DATA_BLOCK DB 1
TITLE =
VERSION : 0.1


  STRUCT
   DB_VAR : BOOL ;	//vorläufige Platzhaltervariable
  END_STRUCT ;
BEGIN
   DB_VAR := FALSE;
END_DATA_BLOCK

DATA_BLOCK "Globaler DB10"
TITLE =
AUTHOR : 'Kleißler'
VERSION : 0.1


  STRUCT
   DB_VAR : INT ;	//vorläufige Platzhaltervariable
   ANALOGWERT : REAL ;	//Analogwert
   ANALOGWERT_BEARB : REAL ;	//Analogwert nach Bearbeitung
   Zykluszeit : REAL ;	//Zykluszeit
   FC_105_Fehlerinfo : WORD ;	//Fehlerinformationen zum FC 105
   FC_106_Fehlerinfo : WORD ;	//Fehlerinformationen zum FC 106
  END_STRUCT ;
BEGIN
   DB_VAR := 0;
   ANALOGWERT := 0.000000e+000;
   ANALOGWERT_BEARB := 0.000000e+000;
   Zykluszeit := 0.000000e+000;
   FC_105_Fehlerinfo := W#16#0;
   FC_106_Fehlerinfo := W#16#0;
END_DATA_BLOCK

FUNCTION "Anlage EIN/AUS" : VOID
TITLE =Allgemeine Funktionen
AUTHOR : 'Kleißler'
VERSION : 0.1

BEGIN
NETWORK
TITLE =HM Anlage EIN_AUS
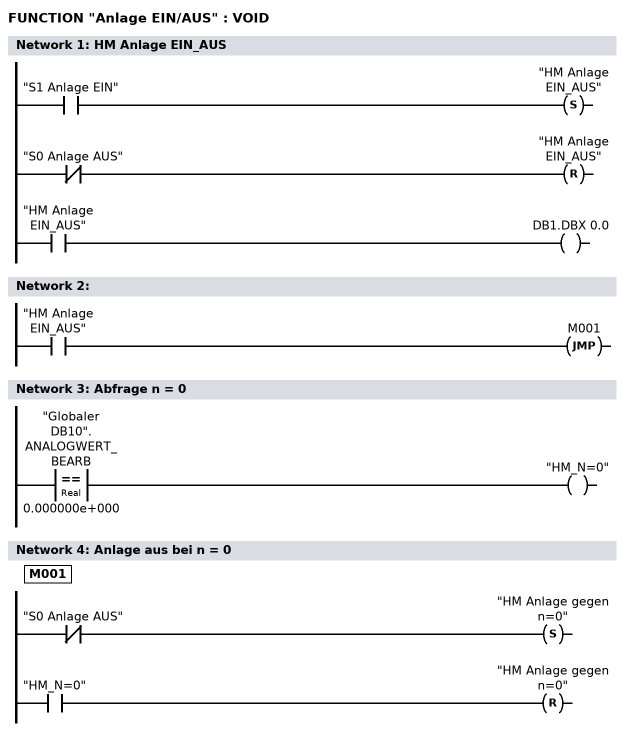
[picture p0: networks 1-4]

      U     "S1 Anlage EIN";
      S     "HM Anlage EIN_AUS";
      UN    "S0 Anlage AUS";
      R     "HM Anlage EIN_AUS";
      U     "HM Anlage EIN_AUS";
      =     DB1.DBX    0.0;
NETWORK
TITLE =

      U     "HM Anlage EIN_AUS";
      SPB   M001;

NETWORK
TITLE =Abfrage n = 0

      L     "Globaler DB10".ANALOGWERT_BEARB;
      L     0.000000e+000;
      ==R   ;
      =     "HM_N=0";
NETWORK
TITLE =Anlage aus bei n = 0

M001: UN    "S0 Anlage AUS";
      S     "HM Anlage gegen n=0";
      U     "HM_N=0";
      R     "HM Anlage gegen n=0";
      NOP   0;
END_FUNCTION

FUNCTION "Ramp_up" : VOID
TITLE =
AUTHOR : 'Kleißler'
VERSION : 0.1

BEGIN
NETWORK
TITLE =Anlage EIN / AUS

      UN    "HM Anlage EIN_AUS";
      SPB   M100;



NETWORK
TITLE =Vergleich Istwert = Sollwert


      L     "Globaler DB10".ANALOGWERT_BEARB;
      L     "Globaler DB10".ANALOGWERT;
      >=R   ;
      SPB   M100;

NETWORK
TITLE =Addition für Rampe


      L     "Globaler DB10".ANALOGWERT_BEARB;
      L     1.000000e+000;
      +R    ;
      T     "Globaler DB10".ANALOGWERT_BEARB;
      NOP   0;

NETWORK
TITLE =Bausteinende


M100: NOP   0;

END_FUNCTION

FUNCTION "Ramp_down" : VOID
TITLE =
AUTHOR : 'Kleißler'
VERSION : 0.1

BEGIN
NETWORK
TITLE =Abfrage n = 0

      L     "Globaler DB10".ANALOGWERT_BEARB;
      L     0.000000e+000;
      <=R   ;
      SPB   M100;




NETWORK
TITLE =Abfrage Anlage EIN

      U     "HM Anlage EIN_AUS";
      SPB   M100;




NETWORK
TITLE =Subtrahiere den Istwert

      L     "Globaler DB10".ANALOGWERT_BEARB;
      L     1.000000e+000;
      -R    ;
      T     "Globaler DB10".ANALOGWERT_BEARB;
      NOP   0;


NETWORK
TITLE =Bausteinende


M100: NOP   0;


END_FUNCTION

FUNCTION "Ramp_down_folgen" : VOID
TITLE =
AUTHOR : 'Kleißler'
VERSION : 0.1

BEGIN
NETWORK
TITLE =Abfrage Anlage ist EIN
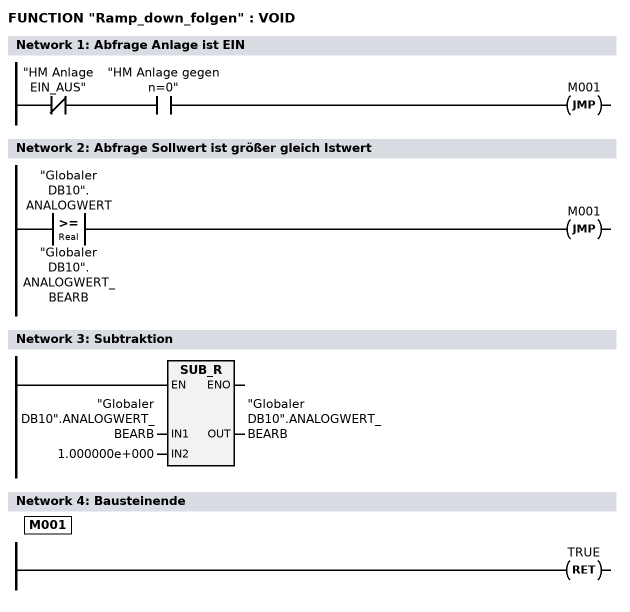
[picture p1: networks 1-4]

      UN    "HM Anlage EIN_AUS";
      U     "HM Anlage gegen n=0";
      SPB   M001;


NETWORK
TITLE =Abfrage Sollwert ist größer gleich Istwert

      L     "Globaler DB10".ANALOGWERT;
      L     "Globaler DB10".ANALOGWERT_BEARB;
      >=R   ;
      SPB   M001;




NETWORK
TITLE =Subtraktion

      L     "Globaler DB10".ANALOGWERT_BEARB;
      L     1.000000e+000;
      -R    ;
      T     "Globaler DB10".ANALOGWERT_BEARB;
      NOP   0;



NETWORK
TITLE =Bausteinende

M001: BE    ;


END_FUNCTION

FUNCTION "Analog einlesen" : VOID
TITLE =Analog einlesen
AUTHOR : 'Kleißler'
VERSION : 0.1

BEGIN
NETWORK
TITLE =Umschaltung Einrich,- Normalbetrieb
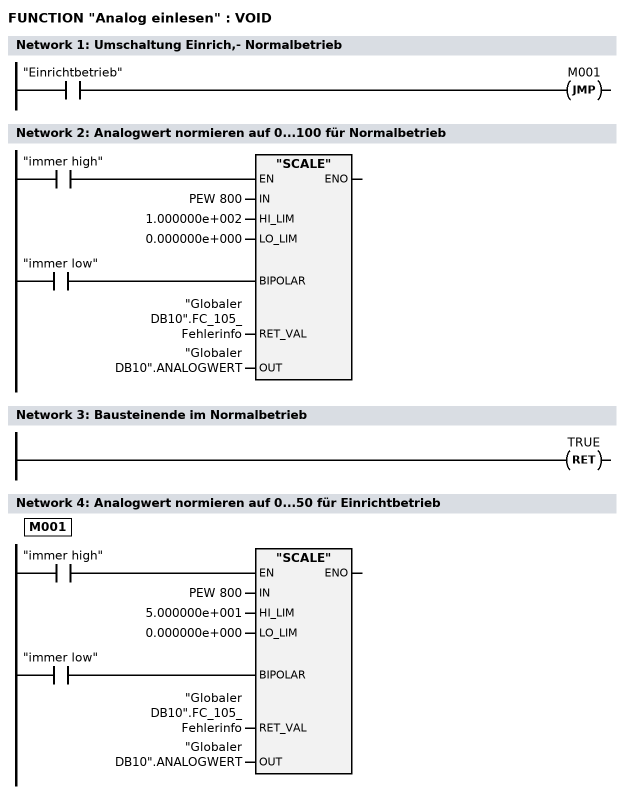
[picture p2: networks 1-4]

      U     "Einrichtbetrieb";
      SPB   M001;

NETWORK
TITLE =Analogwert normieren auf 0...100 für Normalbetrieb

      U     "immer low";
      =     L      0.0;
      BLD   103;
      U     "immer high";
      SPBNB _001;
      CALL "SCALE" (
           IN                       := PEW  800,
           HI_LIM                   := 1.000000e+002,
           LO_LIM                   := 0.000000e+000,
           BIPOLAR                  := L      0.0,
           RET_VAL                  := "Globaler DB10".FC_105_Fehlerinfo,
           OUT                      := "Globaler DB10".ANALOGWERT);
_001: NOP   0;
NETWORK
TITLE =Bausteinende im Normalbetrieb

      BEA   ;
NETWORK
TITLE =Analogwert normieren auf 0...50 für Einrichtbetrieb

M001: U     "immer low";
      =     L      0.0;
      BLD   103;
      U     "immer high";
      SPBNB _002;
      CALL "SCALE" (
           IN                       := PEW  800,
           HI_LIM                   := 5.000000e+001,
           LO_LIM                   := 0.000000e+000,
           BIPOLAR                  := L      0.0,
           RET_VAL                  := "Globaler DB10".FC_105_Fehlerinfo,
           OUT                      := "Globaler DB10".ANALOGWERT);
_002: NOP   0;
END_FUNCTION

FUNCTION "Analog ausgeben" : VOID
TITLE =Analogwert ausgeben
AUTHOR : 'Kleißler'
VERSION : 0.1

BEGIN
NETWORK
TITLE =Analogwert normiert (0...100) ausgeben auf PAW 820

      U     "immer low";
      =     L      0.0;
      BLD   103;
      U     "immer high";
      SPBNB _001;
      CALL "UNSCALE" (
           IN                       := "Globaler DB10".ANALOGWERT_BEARB,
           HI_LIM                   := 1.000000e+002,
           LO_LIM                   := 0.000000e+000,
           BIPOLAR                  := L      0.0,
           RET_VAL                  := "Globaler DB10".FC_106_Fehlerinfo,
           OUT                      := PAW  820);
_001: NOP   0;
END_FUNCTION

FUNCTION "ML steuern" : VOID
TITLE =ML Steuern
AUTHOR : 'Kleißler'
VERSION : 0.1

BEGIN
NETWORK
TITLE =HM n=0 anfahren
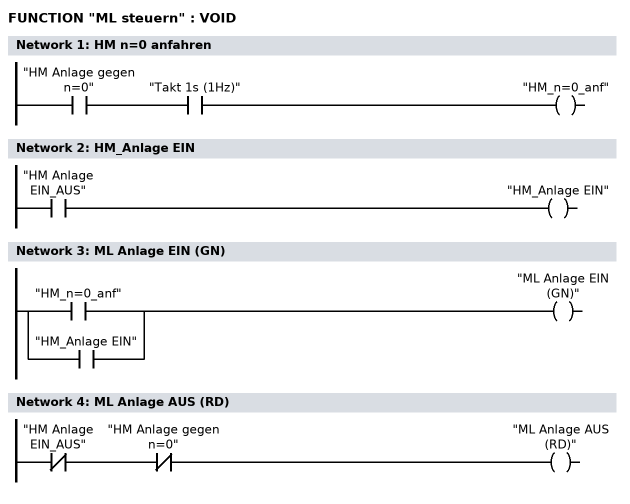
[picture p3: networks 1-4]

      U     "HM Anlage gegen n=0";
      U     "Takt 1s (1Hz)";
      =     "HM_n=0_anf";




NETWORK
TITLE =HM_Anlage EIN

      U     "HM Anlage EIN_AUS";
      =     "HM_Anlage EIN";




NETWORK
TITLE =ML Anlage EIN (GN)

      O     "HM_n=0_anf";
      O     "HM_Anlage EIN";
      =     "ML Anlage EIN (GN)";


NETWORK
TITLE =ML Anlage AUS (RD)

      UN    "HM Anlage EIN_AUS";
      UN    "HM Anlage gegen n=0";
      =     "ML Anlage AUS (RD)";



END_FUNCTION

ORGANIZATION_BLOCK "Programmstruktur"
TITLE = "Main Program Sweep (Cycle)"
AUTHOR : 'Kleißler'
VERSION : 0.1


VAR_TEMP
  OB1_EV_CLASS : BYTE ;	//Bits 0-3 = 1 (Coming event), Bits 4-7 = 1 (Event class 1)
  OB1_SCAN_1 : BYTE ;	//1 (Cold restart scan 1 of OB 1), 3 (Scan 2-n of OB 1)
  OB1_PRIORITY : BYTE ;	//Priority of OB Execution
  OB1_OB_NUMBR : BYTE ;	//1 (Organization block 1, OB1)
  OB1_RESERVED_1 : BYTE ;	//Reserved for system
  OB1_RESERVED_2 : BYTE ;	//Reserved for system
  OB1_PREV_CYCLE : INT ;	//Cycle time of previous OB1 scan (milliseconds)
  OB1_MIN_CYCLE : INT ;	//Minimum cycle time of OB1 (milliseconds)
  OB1_MAX_CYCLE : INT ;	//Maximum cycle time of OB1 (milliseconds)
  OB1_DATE_TIME : DATE_AND_TIME ;	//Date and time OB1 started
END_VAR
BEGIN
NETWORK
TITLE =Hilfsmerker immer low/high
//CLR setzt das VKE auf den Signalzustand "0"
//SET setzt das VKE auf den Signalzustand "1"
      CLR   ;
      =     "immer low";
      SET   ;
      =     "immer high";
NETWORK
TITLE =Aufruf allgemeiner Funktionen

      CALL "Anlage EIN/AUS" ;
      CALL "Analog einlesen" ;
      CALL "Analog ausgeben" ;
      CALL "ML steuern" ;

NETWORK
TITLE =Zeitgesteuerte Aufrufe der Rampenbausteine
//Anstatt des anspringen der Zeitgesteuerten FC´s 2+3+4 über den HW Takt kann auch
//der OB35 (Weckalarm OG) über die HW Projektierung verwendet werden.
      U     "Takt 0,1s (10Hz)";
      FP    "HM Flanke M1.1";
      =     "FM 1.1";

      O     "FM 1.1";
      CC    "Ramp_up";

      O     "FM 1.1";
      CC    "Ramp_down";

      O     "FM 1.1";
      CC    "Ramp_down_folgen";
END_ORGANIZATION_BLOCK

